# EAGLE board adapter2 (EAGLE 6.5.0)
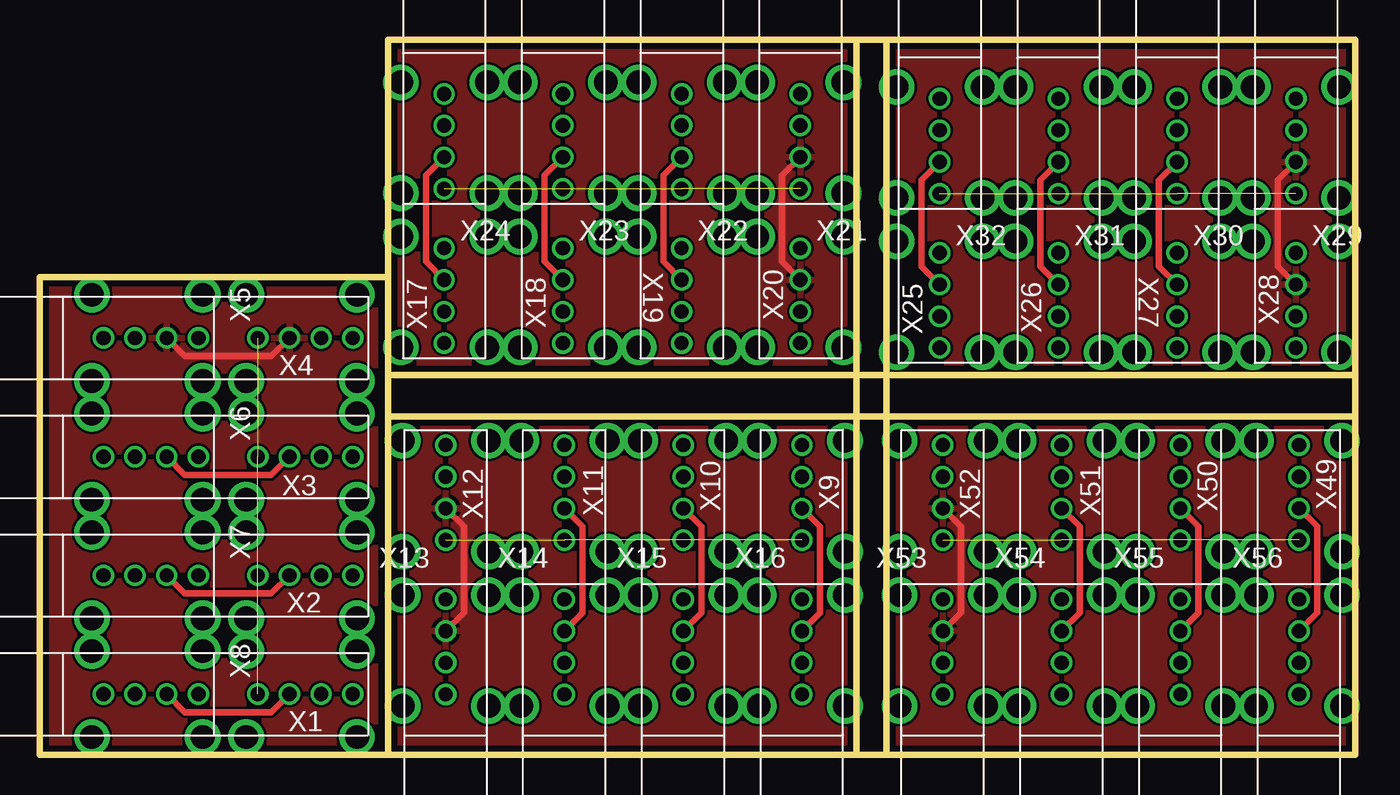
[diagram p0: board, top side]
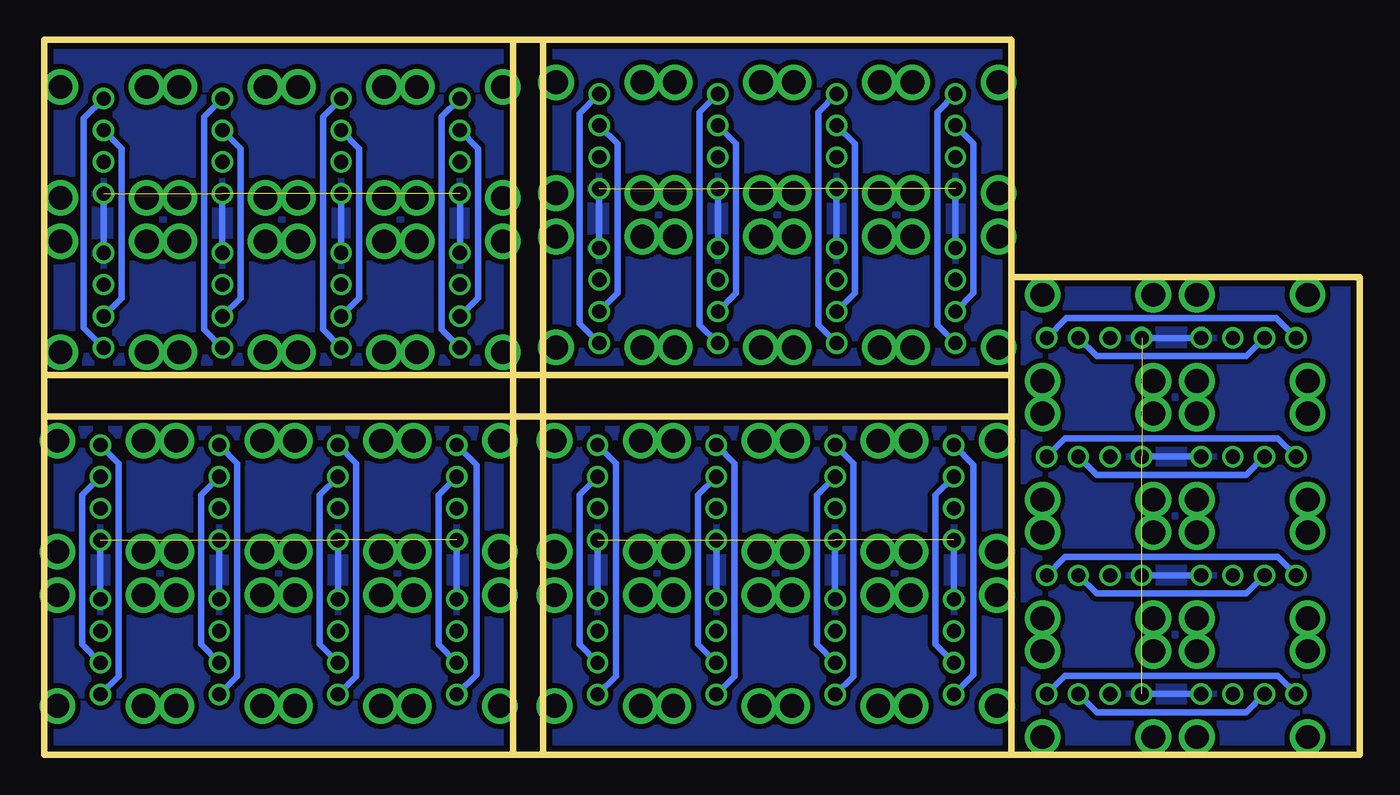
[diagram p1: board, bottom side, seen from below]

Size 83.1 x 45.2 mm. Coordinates in mm from the lower left corner, seen from the top.
Outline: 53.5,0 0,0 0,30.2 22,30.2
Outline: 53.5,0 83.1,0 83.1,21.4
Outline: 83.1,21.4 83.1,24
Outline: 83.1,24 83.1,45.2 53.5,45.2
Outline: 22,0.1 22,21.4
Outline: 22,21.4 22,24
Outline: 22,24 22,30.2
Outline: 51.6,45.2 22,45.2 22,30.2
Outline: 51.6,45.2 53.5,45.2
Outline: 51.6,0.1 51.6,45.2
Outline: 53.5,0 53.5,45.2
Outline: 22,21.4 83.1,21.4
Outline: 83.1,24 22,24
Copper layers (1*16): Top 0.0356mm / dielectric 1.5011mm / Bottom 0.0356mm
Design rules "LaenPCBOrder": minimum track width 6mil, minimum drill 13mil, track to track 6mil, track to pad 6mil, pad to pad 6mil, via to via 6mil, smd to smd 6mil, copper to edge 15mil, drill to drill 6mil, minimum pad ring 7mil, minimum via ring 7mil, stop-mask expansion 3mil, vias tented up to drill 0mil, thermal gap 10mil

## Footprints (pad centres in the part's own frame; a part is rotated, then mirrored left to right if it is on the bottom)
USB-A-HU = drill 0.9: D+ 2.73,0; D- 4.73,0; GND 0.73,0; VBUS 6.73,0 | drill 1.5: P$5 0,2.72; P$6 0,-2.72; P$7 7,2.72; P$8 7,-2.72

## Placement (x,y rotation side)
X1  USB-A-HU  [USB-A-HU]  13.05,3.85 0 top
X2  USB-A-HU  [USB-A-HU]  13.05,11.35 0 top
X3  USB-A-HU  [USB-A-HU]  13.05,18.85 0 top
X4  USB-A-HU  [USB-A-HU]  13.05,26.35 0 top
X5  USB-A-HU  [USB-A-HU]  3.3,26.35 0 top
X6  USB-A-HU  [USB-A-HU]  3.3,18.85 0 top
X7  USB-A-HU  [USB-A-HU]  3.3,11.35 0 top
X8  USB-A-HU  [USB-A-HU]  3.3,3.85 0 top
X9  USB-A-HU  [USB-A-HU]  48.15,12.85 90 top
X10  USB-A-HU  [USB-A-HU]  40.65,12.85 90 top
X11  USB-A-HU  [USB-A-HU]  33.15,12.85 90 top
X12  USB-A-HU  [USB-A-HU]  25.65,12.85 90 top
X13  USB-A-HU  [USB-A-HU]  25.65,3.1 90 top
X14  USB-A-HU  [USB-A-HU]  33.15,3.1 90 top
X15  USB-A-HU  [USB-A-HU]  40.65,3.1 90 top
X16  USB-A-HU  [USB-A-HU]  48.15,3.1 90 top
X17  USB-A-HU  [USB-A-HU]  25.55,32.75 270 top
X18  USB-A-HU  [USB-A-HU]  33.05,32.75 270 top
X19  USB-A-HU  [USB-A-HU]  40.55,32.75 270 top
X20  USB-A-HU  [USB-A-HU]  48.05,32.75 270 top
X21  USB-A-HU  [USB-A-HU]  48.05,42.5 270 top
X22  USB-A-HU  [USB-A-HU]  40.55,42.5 270 top
X23  USB-A-HU  [USB-A-HU]  33.05,42.5 270 top
X24  USB-A-HU  [USB-A-HU]  25.55,42.5 270 top
X25  USB-A-HU  [USB-A-HU]  56.85,32.45 270 top
X26  USB-A-HU  [USB-A-HU]  64.35,32.45 270 top
X27  USB-A-HU  [USB-A-HU]  71.85,32.45 270 top
X28  USB-A-HU  [USB-A-HU]  79.35,32.45 270 top
X29  USB-A-HU  [USB-A-HU]  79.35,42.2 270 top
X30  USB-A-HU  [USB-A-HU]  71.85,42.2 270 top
X31  USB-A-HU  [USB-A-HU]  64.35,42.2 270 top
X32  USB-A-HU  [USB-A-HU]  56.85,42.2 270 top
X49  USB-A-HU  [USB-A-HU]  79.55,12.85 90 top
X50  USB-A-HU  [USB-A-HU]  72.05,12.85 90 top
X51  USB-A-HU  [USB-A-HU]  64.55,12.85 90 top
X52  USB-A-HU  [USB-A-HU]  57.05,12.85 90 top
X53  USB-A-HU  [USB-A-HU]  57.05,3.1 90 top
X54  USB-A-HU  [USB-A-HU]  64.55,3.1 90 top
X55  USB-A-HU  [USB-A-HU]  72.05,3.1 90 top
X56  USB-A-HU  [USB-A-HU]  79.55,3.1 90 top

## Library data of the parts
X1-X32 X49-X56 = con-usb

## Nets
DM1: X4.D- X5.D+
DM2: X12.D- X13.D+
DM3: X20.D- X21.D+
DM4: X28.D- X29.D+
DM7: X52.D- X53.D+
DP1: X4.D+ X5.D-
DP2: X12.D+ X13.D-
DP3: X20.D+ X21.D-
DP4: X28.D+ X29.D-
DP7: X52.D+ X53.D-
GND: X1.GND X2.GND X3.GND X4.GND X5.VBUS X6.VBUS X7.VBUS X8.VBUS
GND1: X17.GND X18.GND X19.GND X20.GND X21.VBUS X22.VBUS X23.VBUS X24.VBUS
GND4: X9.GND X10.GND X11.GND X12.GND X13.VBUS X14.VBUS X15.VBUS X16.VBUS
GND7: X49.GND X50.GND X51.GND X52.GND X53.VBUS X54.VBUS X55.VBUS X56.VBUS
GND10: X25.GND X26.GND X27.GND X28.GND X29.VBUS X30.VBUS X31.VBUS X32.VBUS
N$1: X1.VBUS X8.GND
N$2: X10.VBUS X15.GND
N$3: X3.D+ X6.D-
N$4: X3.D- X6.D+
N$5: X11.VBUS X14.GND
N$6: X2.D+ X7.D-
N$7: X2.D- X7.D+
N$8: X12.VBUS X13.GND
N$9: X1.D+ X8.D-
N$10: X2.VBUS X7.GND
N$11: X3.VBUS X6.GND
N$12: X4.VBUS X5.GND
N$13: X1.D- X8.D+
N$14: X9.VBUS X16.GND
N$15: X11.D+ X14.D-
N$16: X11.D- X14.D+
N$17: X10.D+ X15.D-
N$18: X10.D- X15.D+
N$19: X9.D+ X16.D-
N$20: X9.D- X16.D+
N$21: X18.VBUS X23.GND
N$22: X19.VBUS X22.GND
N$23: X20.VBUS X21.GND
N$24: X17.VBUS X24.GND
N$25: X19.D+ X22.D-
N$26: X19.D- X22.D+
N$27: X18.D+ X23.D-
N$28: X18.D- X23.D+
N$29: X17.D+ X24.D-
N$30: X17.D- X24.D+
N$31: X26.VBUS X31.GND
N$32: X27.VBUS X30.GND
N$33: X28.VBUS X29.GND
N$34: X25.VBUS X32.GND
N$35: X27.D+ X30.D-
N$36: X27.D- X30.D+
N$37: X26.D+ X31.D-
N$38: X26.D- X31.D+
N$39: X25.D+ X32.D-
N$40: X25.D- X32.D+
N$61: X50.VBUS X55.GND
N$62: X51.VBUS X54.GND
N$63: X52.VBUS X53.GND
N$64: X49.VBUS X56.GND
N$65: X51.D+ X54.D-
N$66: X51.D- X54.D+
N$67: X50.D+ X55.D-
N$68: X50.D- X55.D+
N$69: X49.D+ X56.D-
N$70: X49.D- X56.D+

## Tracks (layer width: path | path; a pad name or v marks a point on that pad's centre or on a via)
DM1
  Bottom 0.406: X4.D- 16.63,25.2 7.18,25.2 X5.D+
DM2
  Bottom 0.406: X12.D- 26.8,16.43 26.8,6.98 X13.D+
DM3
  Bottom 0.406: X20.D- 46.9,29.17 46.9,38.62 X21.D+
DM4
  Bottom 0.406: X28.D- 78.2,28.87 78.2,38.32 X29.D+
DM7
  Bottom 0.406: X52.D- 58.2,16.43 58.2,6.98 X53.D+
DP1
  Top 0.406: X5.D- 9.18,25.2 14.63,25.2 X4.D+
  pour Top: 0.6,29.7 0.6,0.6 21.2,0.6 21.2,29.7
DP2
  Top 0.406: X13.D- 26.8,8.98 26.8,14.43 X12.D+
  pour Top: 22.3,0.4 51.4,0.4 51.4,21 22.3,21 22.3,0.5
DP3
  Top 0.406: X21.D- 46.9,36.62 46.9,31.17 X20.D+
  pour Top: 51.4,45.2 22.3,45.2 22.3,24.6 51.4,24.6
DP4
  Top 0.406: X29.D- 78.2,36.32 78.2,30.87 X28.D+
  pour Top: 82.7,44.9 53.6,44.9 53.6,24.3 82.7,24.3 82.7,44.8
DP7
  Top 0.406: X53.D- 58.2,8.98 58.2,14.43 X52.D+
  pour Top: 53.7,0.4 82.8,0.4 82.8,21 53.7,21 53.7,0.5
GND  (3 unrouted)
  Bottom 0.406: X4.GND X5.VBUS | X3.GND X6.VBUS | X2.GND X7.VBUS | X1.GND X8.VBUS
  pour Bottom (isolate 0.305): 0.5,29.7 0.5,0.6 21.3,0.6 21.3,29.7
GND1  (3 unrouted)
  Bottom 0.406: X20.GND X21.VBUS | X19.GND X22.VBUS | X18.GND X23.VBUS | X17.GND X24.VBUS
  pour Bottom (isolate 0.305): 51.4,45.3 22.3,45.3 22.3,24.5 51.4,24.5
GND4  (3 unrouted)
  Bottom 0.406: X12.GND X13.VBUS | X11.GND X14.VBUS | X10.GND X15.VBUS | X9.GND X16.VBUS
  pour Bottom (isolate 0.305): 22.3,0.3 51.4,0.3 51.4,21.1 22.3,21.1
GND7  (3 unrouted)
  Bottom 0.406: X52.GND X53.VBUS | X51.GND X54.VBUS | X50.GND X55.VBUS | X49.GND X56.VBUS
  pour Bottom (isolate 0.305): 53.7,0.3 82.8,0.3 82.8,21.1 53.7,21.1
GND10  (3 unrouted)
  Bottom 0.406: X28.GND X29.VBUS | X27.GND X30.VBUS | X26.GND X31.VBUS | X25.GND X32.VBUS
  pour Bottom (isolate 0.305): 82.7,45 53.6,45 53.6,24.2 82.7,24.2
N$1
  Bottom 0.406: X8.GND 5.18,5 18.63,5 X1.VBUS
N$2
  Bottom 0.406: X15.GND 39.5,4.98 39.5,18.43 X10.VBUS
N$3
  Top 0.406: X6.D- 9.18,17.7 14.63,17.7 X3.D+
N$4
  Bottom 0.406: X6.D+ 7.18,17.7 16.63,17.7 X3.D-
N$5
  Bottom 0.406: X11.VBUS 32,18.43 32,4.98 X14.GND
N$6
  Top 0.406: X7.D- 9.18,10.2 14.63,10.2 X2.D+
N$7
  Bottom 0.406: X2.D- 16.63,10.2 7.18,10.2 X7.D+
N$8
  Bottom 0.406: X12.VBUS 24.4,18.33 24.4,5.08 X13.GND
N$9
  Top 0.406: X8.D- 9.18,2.7 14.63,2.7 X1.D+
N$10
  Bottom 0.406: X7.GND 5.18,12.5 18.63,12.5 X2.VBUS
N$11
  Bottom 0.406: X3.VBUS 18.63,20 5.18,20 X6.GND
N$12
  Bottom 0.406: X4.VBUS 18.53,27.6 5.28,27.6 X5.GND
N$13
  Bottom 0.406: X1.D- 16.63,2.7 7.18,2.7 X8.D+
N$14
  Bottom 0.406: X16.GND 47,4.98 47,18.43 X9.VBUS
N$15
  Top 0.406: X14.D- 34.3,8.98 34.3,14.43 X11.D+
N$16
  Bottom 0.406: X14.D+ 34.3,6.98 34.3,16.43 X11.D-
N$17
  Top 0.406: X15.D- 41.8,8.98 41.8,14.43 X10.D+
N$18
  Bottom 0.406: X10.D- 41.8,16.43 41.8,6.98 X15.D+
N$19
  Top 0.406: X16.D- 49.3,8.98 49.3,14.43 X9.D+
N$20
  Bottom 0.406: X9.D- 49.3,16.43 49.3,6.98 X16.D+
N$21
  Bottom 0.406: X23.GND 34.2,40.62 34.2,27.17 X18.VBUS
N$22
  Bottom 0.406: X19.VBUS 41.7,27.17 41.7,40.62 X22.GND
N$23
  Bottom 0.406: X20.VBUS 49.3,27.27 49.3,40.52 X21.GND
N$24
  Bottom 0.406: X24.GND 26.7,40.62 26.7,27.17 X17.VBUS
N$25
  Top 0.406: X22.D- 39.4,36.62 39.4,31.17 X19.D+
N$26
  Bottom 0.406: X22.D+ 39.4,38.62 39.4,29.17 X19.D-
N$27
  Top 0.406: X23.D- 31.9,36.62 31.9,31.17 X18.D+
N$28
  Bottom 0.406: X18.D- 31.9,29.17 31.9,38.62 X23.D+
N$29
  Top 0.406: X24.D- 24.4,36.62 24.4,31.17 X17.D+
N$30
  Bottom 0.406: X17.D- 24.4,29.17 24.4,38.62 X24.D+
N$31
  Bottom 0.406: X31.GND 65.5,40.32 65.5,26.87 X26.VBUS
N$32
  Bottom 0.406: X27.VBUS 73,26.87 73,40.32 X30.GND
N$33
  Bottom 0.406: X28.VBUS 80.6,26.97 80.6,40.22 X29.GND
N$34
  Bottom 0.406: X32.GND 58,40.32 58,26.87 X25.VBUS
N$35
  Top 0.406: X30.D- 70.7,36.32 70.7,30.87 X27.D+
N$36
  Bottom 0.406: X30.D+ 70.7,38.32 70.7,28.87 X27.D-
N$37
  Top 0.406: X31.D- 63.2,36.32 63.2,30.87 X26.D+
N$38
  Bottom 0.406: X26.D- 63.2,28.87 63.2,38.32 X31.D+
N$39
  Top 0.406: X32.D- 55.7,36.32 55.7,30.87 X25.D+
N$40
  Bottom 0.406: X25.D- 55.7,28.87 55.7,38.32 X32.D+
N$61
  Bottom 0.406: X55.GND 70.9,4.98 70.9,18.43 X50.VBUS
N$62
  Bottom 0.406: X51.VBUS 63.4,18.43 63.4,4.98 X54.GND
N$63
  Bottom 0.406: X52.VBUS 55.8,18.33 55.8,5.08 X53.GND
N$64
  Bottom 0.406: X56.GND 78.4,4.98 78.4,18.43 X49.VBUS
N$65
  Top 0.406: X54.D- 65.7,8.98 65.7,14.43 X51.D+
N$66
  Bottom 0.406: X54.D+ 65.7,6.98 65.7,16.43 X51.D-
N$67
  Top 0.406: X55.D- 73.2,8.98 73.2,14.43 X50.D+
N$68
  Bottom 0.406: X50.D- 73.2,16.43 73.2,6.98 X55.D+
N$69
  Top 0.406: X56.D- 80.7,8.98 80.7,14.43 X49.D+
N$70
  Bottom 0.406: X49.D- 80.7,16.43 80.7,6.98 X56.D+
